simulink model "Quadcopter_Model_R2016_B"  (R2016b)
settings: Solver=VariableStepAuto  StartTime=0.0  StopTime=20  RelTol=1e-3
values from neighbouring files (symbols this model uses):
  g = 9.81    [modelParameters.m]
  If = 0.511    [modelParameters.m]
  Jreq = 4.2012e-05    [modelParameters.m]
  Jxx = 0.0218    [modelParameters.m]
  Jyy = 0.0277    [modelParameters.m]
  Jzz = 0.0332    [modelParameters.m]
  Kd = 1.8087e-07    [modelParameters.m]
  Kq = 96.3422    [modelParameters.m]
  Kt = 8.1558*10^-6    (= 8.1558e-06)    [modelParameters.m]
  Kv = 96.3422    [modelParameters.m]
  m = 1.19    [modelParameters.m]
  Pmax = 0.80    (= 0.8)    [modelParameters.m]
  Pmin = 0.40    (= 0.4)    [modelParameters.m]
  rhx = 0.016    [modelParameters.m]
  rhy = 0.016    [modelParameters.m]
  rhz = 0.003    [modelParameters.m]
  Rm = 0.2308    [modelParameters.m]
  Vb = 11.1    [modelParameters.m]
libraries: vrlib x2, simulink x2

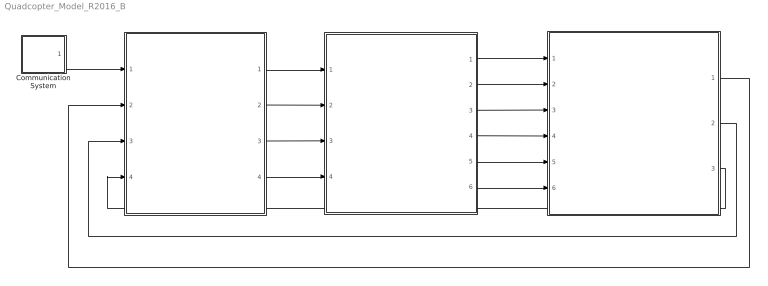
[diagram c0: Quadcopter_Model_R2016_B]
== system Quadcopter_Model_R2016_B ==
  " " : Subsystem
  "        " : Subsystem
  " " : Subsystem
  Communication System : Subsystem
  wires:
  " "/1(Rotor 0 Duty Cycle) -> " "/1(Rotor 0 Duty Cycle)
  "        "/2(euler_rates) -> " "/3(euler_rates)
  "        "/1(euler_angles_filtered) -> " "/2(euler_angles_filtered)
  Communication System/1(setpoints) -> " "/1(setpoints)
  " "/2(Rotor 1 Duty Cycle) -> " "/2(Rotor 1 Duty Cycle)
  " "/3(Rotor 2 Duty Cycle) -> " "/3(Rotor 2 Duty Cycle)
  " "/4(Rotor 3 Duty Cycle) -> " "/4(Rotor 3 Duty Cycle)
  " "/1(B_omega) -> "        "/1(B_Omega)
  " "/2(euler_angles) -> "        "/2(euler_angles)
  " "/3(B_vo) -> "        "/3(B_vo)
  " "/4(E_ro) -> "        "/4(E_ro)
  " "/5(B_vo_dot) -> "        "/5(B_vo_dot)
  " "/6(B_g) -> "        "/6(B_g)
  "        "/3(current_position) -> " "/4(current_position)

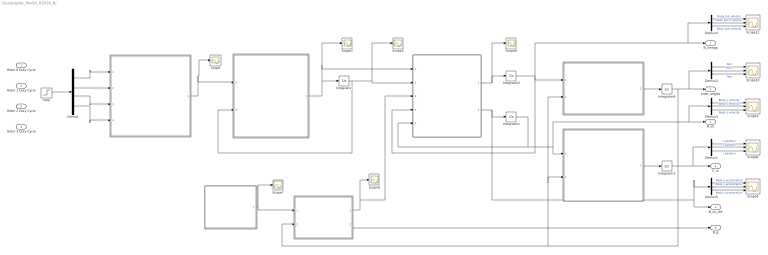
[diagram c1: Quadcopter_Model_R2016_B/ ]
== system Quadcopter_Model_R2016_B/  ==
  Rotor 0 Duty Cycle : Inport
  Rotor 1 Duty Cycle : Inport  Port=2
  Rotor 2 Duty Cycle : Inport  Port=3
  Rotor 3 Duty Cycle : Inport  Port=4
  " " : MATLAB Function  TreatAsAtomicUnit=on
  " " : MATLAB Function  TreatAsAtomicUnit=on
  " " : MATLAB Function  TreatAsAtomicUnit=on
  " " : MATLAB Function  TreatAsAtomicUnit=on
  " " : MATLAB Function  TreatAsAtomicUnit=on
  " " : MATLAB Function  TreatAsAtomicUnit=on
  " " : MATLAB Function  TreatAsAtomicUnit=on
  Demux : Demux
  Demux{1..5} (5 alike) : Demux  Outputs=3
  Integrator{,1..3} (4 alike) : Integrator
  Integrator4 : Integrator  ContinuousStateAttributes=['phi' 'theta' 'psi']
  Scope{,1..2,7..9} (6 alike) : Scope
  Scope{3..4,6,10..11} (5 alike) : Scope  NumInputPorts=3
  Step : Step  Before=68.25*ones(4,1)  After=[ 68.25; 69.25; 69.25; 68.25 ]  SampleTime=0
  B_omega : Outport
  euler_angles : Outport  Port=2
  B_vo : Outport  Port=3
  E_ro : Outport  Port=4
  B_vo_dot : Outport  Port=5
  B_g : Outport  Port=6
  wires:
  " "/1(Vb_eff) -> Scope/1, " "/1(Vb_eff)
  " "/1(angular_acceleration) -> Integrator/1, Scope1/1, " "/1(angular_acceleration)
  Integrator/1 -> Scope2/1, " "/2(angular_velocity), " "/2(angular_velocity)
  " "/1(B_omega_dot) -> Scope9/1, Integrator2/1
  " "/2(B_vo_dot) -> Demux5/1, B_vo_dot/1, Integrator1/1
  Integrator2/1 -> B_omega/1, Demux4/1, " "/4(B_omega), " "/1(B_omega)
  " "/1(euler_rates) -> Integrator4/1
  " "/1(E_Fg) -> Scope7/1, " "/1(E_Fg)
  " "/1(E_ro) -> Integrator3/1
  Integrator3/1 -> Demux1/1, E_ro/1
  " "/1(B_Fg) -> Scope8/1, " "/3(B_Fg)
  " "/2(B_g) -> B_g/1
  Demux/1 -> " "/1(rotor_0_duty_cycle)
  Demux/2 -> " "/2(rotor_1_duty_cycle)
  Demux/3 -> " "/3(rotor_2_duty_cycle)
  Demux/4 -> " "/4(rotor_3_duty_cycle)
  Step/1 -> Demux/1
  Demux1/2 -> Scope6/2  "y position"
  Demux1/1 -> Scope6/1  "x position"
  Demux1/3 -> Scope6/3  "z position"
  Integrator4/1 -> Demux2/1, euler_angles/1, " "/2(euler_angles), " "/2(euler_angles), " "/2(euler_angles)
  Demux2/2 -> Scope10/2  "Pitch"
  Demux2/1 -> Scope10/1  "Roll"
  Demux2/3 -> Scope10/3  "Yaw"
  Demux4/2 -> Scope11/2  "Body pitch velocity"
  Demux4/1 -> Scope11/1  "Body roll velocity"
  Demux4/3 -> Scope11/3  "Body yaw velocity"
  Demux3/2 -> Scope3/2  "Body y velocity"
  Demux3/1 -> Scope3/1  "Body x velocity"
  Demux3/3 -> Scope3/3  "Body z velocity"
  Demux5/2 -> Scope4/2  "Body y acceleration"
  Demux5/1 -> Scope4/1  "Body x acceleration"
  Demux5/3 -> Scope4/3  "Body z acceleration"
  Integrator1/1 -> " "/5(B_vo), " "/1(B_vo), Demux3/1, B_vo/1

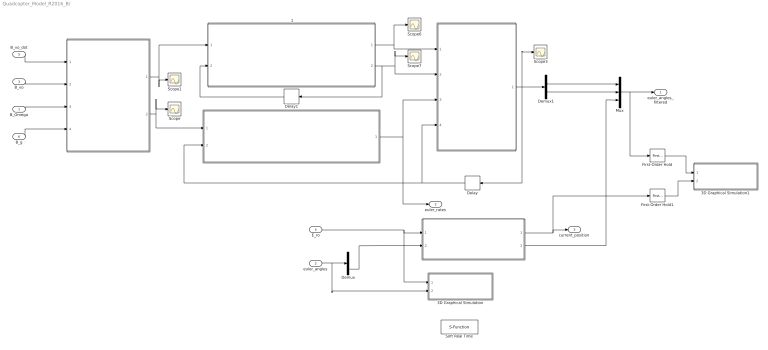
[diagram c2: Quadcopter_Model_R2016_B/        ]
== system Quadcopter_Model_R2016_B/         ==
  B_Omega : Inport
  euler_angles : Inport  Port=2
  B_vo : Inport  Port=3
  E_ro : Inport  Port=4
  B_vo_dot : Inport  Port=5
  B_g : Inport  Port=6
  " " : MATLAB Function  TreatAsAtomicUnit=on
  " " : Subsystem
  " " : MATLAB Function  TreatAsAtomicUnit=on
  " 1" : MATLAB Function  TreatAsAtomicUnit=on
  " " : Subsystem
  3D Graphical Simulation : Subsystem  Commented=on
  3D Graphical Simulation1 : Subsystem
  Delay : Delay  DelayLength=1  InitialCondition=0
  Delay1 : Delay  DelayLength=1  InitialCondition=0
  Demux : Demux  Outputs=3
  Demux1 : Demux  Outputs=2
  First-Order Hold : simulink/Discrete/First-Order Hold  DisableCoverage=on  Ts=6.1e-3
  First-Order Hold1 : simulink/Discrete/First-Order Hold  DisableCoverage=on  Ts=6.1e-3
  Mux : Mux  Inputs=3
  Scope{,1,3,6..7} (5 alike) : Scope
  Soft Real Time : S-Function  Commented=on  FunctionName=sfun_time  Parameters=x  SFunctionDeploymentMode=off  EnableBusSupport=off
  euler_angles_filtered : Outport
  euler_rates : Outport  Port=2
  current_position : Outport  Port=3
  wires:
  " "/1(accelerometer) -> " 1"/1(accel_reading), Scope1/1
  " "/2(gyroscope) -> Scope/1, " "/1(gyro_reading)
  B_vo_dot/1 -> " "/1(B_vo_dot)
  B_vo/1 -> " "/2(B_vo)
  B_Omega/1 -> " "/3(B_Omega)
  B_g/1 -> " "/4(B_g)
  " 1"/2(accel_roll) -> Delay1/1, " "/2(accel_roll), Scope7/1
  " 1"/1(accel_pitch) -> " "/1(accel_pitch), Scope6/1
  " "/1(euler_rates_IMU) -> euler_rates/1, " "/3(euler_angles_gyro)
  Delay/1 -> " "/4(prev_euler_angles_IMU), " "/2(euler_angles_IMU)
  Delay1/1 -> " 1"/2(accel_roll_prev)
  euler_angles/1 -> 3D Graphical Simulation/2(Euler Angles), Demux/1
  " "/1(euler_angles_IMU) -> Demux1/1, Delay/1, Scope3/1
  First-Order Hold/1 -> 3D Graphical Simulation1/1("Euler Angles ")
  E_ro/1 -> 3D Graphical Simulation/1(Displacement), " "/1(E_ro)
  Demux/3 -> " "/2(yaw)
  First-Order Hold1/1 -> 3D Graphical Simulation1/2(Displacement)
  Demux1/1 -> Mux/1
  Demux1/2 -> Mux/2
  " "/2(yaw_camera) -> Mux/3
  Mux/1 -> First-Order Hold/1, euler_angles_filtered/1
  " "/1(E_ro_camera) -> First-Order Hold1/1, current_position/1

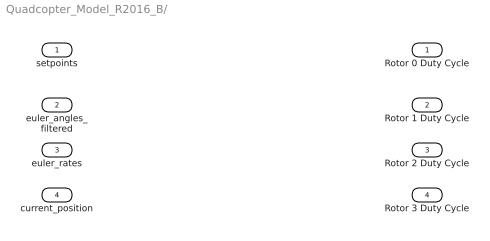
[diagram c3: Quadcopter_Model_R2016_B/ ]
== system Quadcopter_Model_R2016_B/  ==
  setpoints : Inport
  euler_angles_filtered : Inport  Port=2
  euler_rates : Inport  Port=3
  current_position : Inport  Port=4
  Rotor 0 Duty Cycle : Outport
  Rotor 1 Duty Cycle : Outport  Port=2
  Rotor 2 Duty Cycle : Outport  Port=3
  Rotor 3 Duty Cycle : Outport  Port=4

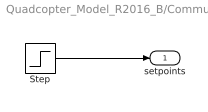
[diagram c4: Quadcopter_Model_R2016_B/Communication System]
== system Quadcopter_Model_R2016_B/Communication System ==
  Step : Step  Before=zeros(4,1)  After=[0; 0; 0; 0]  SampleTime=0
  setpoints : Outport
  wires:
  Step/1 -> setpoints/1

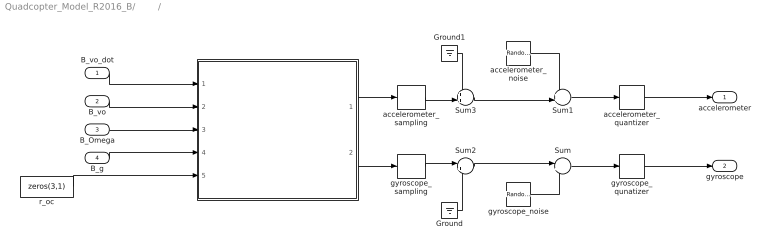
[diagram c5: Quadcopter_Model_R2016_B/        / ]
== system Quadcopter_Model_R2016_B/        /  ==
  B_vo_dot : Inport
  B_vo : Inport  Port=2
  B_Omega : Inport  Port=3
  B_g : Inport  Port=4
  " " : MATLAB Function  TreatAsAtomicUnit=on
  Ground : Ground
  Ground1 : Ground
  Sum : Sum  Inputs=|++
  Sum1 : Sum  Inputs=++|
  Sum2 : Sum  Inputs=|++
  Sum3 : Sum  Inputs=++|
  accelerometer_noise : RandomNumber  Mean=zeros(3,1)  Variance=[ 3e-7 ; 3.3e-7 ; 7.2e-7 ]  Seed=[0,1,2]  SampleTime=6.1e-3
  accelerometer_quantizer : Quantizer  QuantizationInterval=2.4400e-04
  accelerometer_sampling : ZeroOrderHold  SampleTime=6.1e-3
  gyroscope_noise : RandomNumber  Mean=zeros(3,1)  Variance=[ 2.2e-8 ; 1.1e-7 ; 2.4e-8 ]  Seed=[0,1,2]  SampleTime=6.1e-3
  gyroscope_qunatizer : Quantizer  QuantizationInterval=1.1e-3
  gyroscope_sampling : ZeroOrderHold  SampleTime=6.1e-3
  r_oc : Constant  Value=zeros(3,1)
  accelerometer : Outport
  gyroscope : Outport  Port=2
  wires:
  gyroscope_qunatizer/1 -> gyroscope/1
  accelerometer_quantizer/1 -> accelerometer/1
  accelerometer_noise/1 -> Sum1/1
  Sum/1 -> gyroscope_qunatizer/1
  Sum2/1 -> Sum/1
  Sum3/1 -> Sum1/2
  " "/2(gyroReading) -> gyroscope_sampling/1
  gyroscope_noise/1 -> Sum/2
  " "/1(accelReading) -> accelerometer_sampling/1
  Sum1/1 -> accelerometer_quantizer/1
  gyroscope_sampling/1 -> Sum2/1
  accelerometer_sampling/1 -> Sum3/2
  Ground/1 -> Sum2/2
  Ground1/1 -> Sum3/1
  B_vo_dot/1 -> " "/1(B_vo_dot)
  B_vo/1 -> " "/2(B_vo)
  B_Omega/1 -> " "/3(B_Omega)
  B_g/1 -> " "/4(B_g)
  r_oc/1 -> " "/5(r_oc)

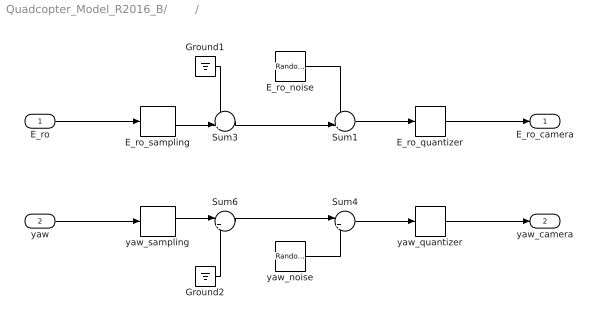
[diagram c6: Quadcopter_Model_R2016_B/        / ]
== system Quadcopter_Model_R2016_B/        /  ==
  E_ro : Inport
  yaw : Inport  Port=2
  E_ro_noise : RandomNumber  Mean=zeros(3,1)  Variance=[ 7.9664e-10 ; 1.1928e-10 ; 5.0636e-10 ]  Seed=[0,1,2]  SampleTime=6.1e-3
  E_ro_quantizer : Quantizer  QuantizationInterval=2.4400e-04
  E_ro_sampling : ZeroOrderHold  SampleTime=6.1e-3
  Ground1 : Ground
  Ground2 : Ground
  Sum1 : Sum  Inputs=++|
  Sum3 : Sum  Inputs=++|
  Sum4 : Sum  Inputs=|++
  Sum6 : Sum  Inputs=|++
  yaw_noise : RandomNumber  Variance=1.0783e-9  SampleTime=6.1e-3
  yaw_quantizer : Quantizer  QuantizationInterval=1.1e-3
  yaw_sampling : ZeroOrderHold  SampleTime=6.1e-3
  E_ro_camera : Outport
  yaw_camera : Outport  Port=2
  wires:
  E_ro_quantizer/1 -> E_ro_camera/1
  E_ro_noise/1 -> Sum1/1
  Sum3/1 -> Sum1/2
  Sum1/1 -> E_ro_quantizer/1
  E_ro_sampling/1 -> Sum3/2
  Ground1/1 -> Sum3/1
  yaw_quantizer/1 -> yaw_camera/1
  Sum4/1 -> yaw_quantizer/1
  Sum6/1 -> Sum4/1
  yaw_noise/1 -> Sum4/2
  yaw_sampling/1 -> Sum6/1
  Ground2/1 -> Sum6/2
  yaw/1 -> yaw_sampling/1
  E_ro/1 -> E_ro_sampling/1

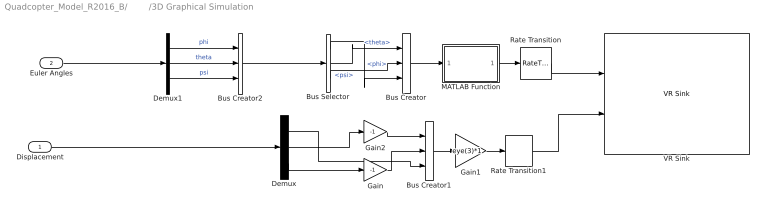
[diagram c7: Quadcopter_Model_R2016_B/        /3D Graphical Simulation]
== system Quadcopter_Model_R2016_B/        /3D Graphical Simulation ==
  Displacement : Inport
  Euler Angles : Inport  Port=2
  Bus Creator : BusCreator  Inputs=3
  Bus Creator1 : BusCreator  Inputs=3
  Bus Creator2 : BusCreator  Inputs=3
  Bus Selector : BusSelector  OutputSignals=phi,theta,psi
  Demux : Demux  Outputs=3
  Demux1 : Demux  Outputs=3
  Gain : Gain  Gain=-1
  Gain1 : Gain  Gain=eye(3)*1  Multiplication=Matrix(K*u)
  Gain2 : Gain  Gain=-1
  MATLAB Function : MATLAB Function  TreatAsAtomicUnit=on
  Rate Transition : RateTransition  OutPortSampleTime=0.06
  Rate Transition1 : RateTransition  OutPortSampleTime=0.06
  VR Sink : vrlib/VR Sink  InstantiateOnLoad=on  SampleTime=-1  ViewEnable=on  RemoteChange=off  RemoteView=off  FieldsWritten=Helicopter.rotation.4.1.1.double#Helicopter.translation.3.1.1.double  WorldFileName=quadrotor_world_ucart.wrl  AutoView=on  VideoDimensions=[]  AllowVariableSize=off
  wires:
  Displacement/1 -> Demux/1
  Bus Creator2/1 -> Bus Selector/1
  Demux/1 -> Bus Creator1/3
  Gain/1 -> Bus Creator1/2
  Gain2/1 -> Bus Creator1/1
  Rate Transition1/1 -> VR Sink/2
  Rate Transition/1 -> VR Sink/1
  Demux/3 -> Gain/1
  Demux/2 -> Gain2/1
  Bus Creator1/1 -> Gain1/1
  Bus Selector/1 -> Bus Creator/3  "<phi>"
  Bus Selector/3 -> Bus Creator/2  "<psi>"
  Bus Selector/2 -> Bus Creator/1  "<theta>"
  Gain1/1 -> Rate Transition1/1
  Demux1/3 -> Bus Creator2/3  "psi"
  Demux1/2 -> Bus Creator2/2  "theta"
  Demux1/1 -> Bus Creator2/1  "phi"
  Euler Angles/1 -> Demux1/1
  Bus Creator/1 -> MATLAB Function/1(u)
  MATLAB Function/1(y) -> Rate Transition/1

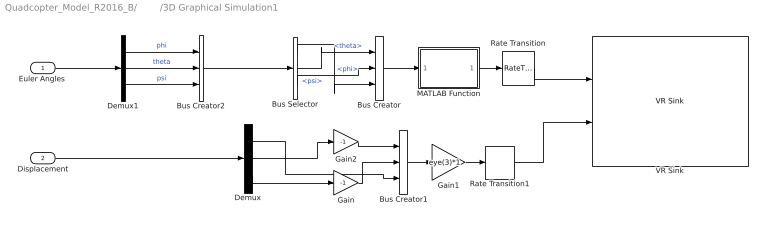
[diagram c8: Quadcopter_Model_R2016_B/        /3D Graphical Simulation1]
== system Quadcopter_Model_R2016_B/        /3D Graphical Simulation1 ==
  "Euler Angles " : Inport
  Displacement : Inport  Port=2
  Bus Creator : BusCreator  Inputs=3
  Bus Creator1 : BusCreator  Inputs=3
  Bus Creator2 : BusCreator  Inputs=3
  Bus Selector : BusSelector  OutputSignals=phi,theta,psi
  Demux : Demux  Outputs=3
  Demux1 : Demux  Outputs=3
  Gain : Gain  Gain=-1
  Gain1 : Gain  Gain=eye(3)*1  Multiplication=Matrix(K*u)
  Gain2 : Gain  Gain=-1
  MATLAB Function : MATLAB Function  TreatAsAtomicUnit=on
  Rate Transition : RateTransition  OutPortSampleTime=0.06
  Rate Transition1 : RateTransition  OutPortSampleTime=0.06
  VR Sink : vrlib/VR Sink  InstantiateOnLoad=on  SampleTime=-1  ViewEnable=on  RemoteChange=off  RemoteView=off  FieldsWritten=Helicopter.rotation.4.1.1.double#Helicopter.translation.3.1.1.double  WorldFileName=quadrotor_world_ucart.wrl  AutoView=on  VideoDimensions=[]  AllowVariableSize=off
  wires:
  Bus Creator2/1 -> Bus Selector/1
  Demux/1 -> Bus Creator1/3
  Gain/1 -> Bus Creator1/2
  Gain2/1 -> Bus Creator1/1
  Rate Transition1/1 -> VR Sink/2
  Rate Transition/1 -> VR Sink/1
  Demux/3 -> Gain/1
  Demux/2 -> Gain2/1
  Bus Creator1/1 -> Gain1/1
  Bus Selector/1 -> Bus Creator/3  "<phi>"
  Bus Selector/3 -> Bus Creator/2  "<psi>"
  Bus Selector/2 -> Bus Creator/1  "<theta>"
  Gain1/1 -> Rate Transition1/1
  Demux1/3 -> Bus Creator2/3  "psi"
  Demux1/2 -> Bus Creator2/2  "theta"
  Demux1/1 -> Bus Creator2/1  "phi"
  Bus Creator/1 -> MATLAB Function/1(u)
  MATLAB Function/1(y) -> Rate Transition/1
  Displacement/1 -> Demux/1
  "Euler Angles "/1 -> Demux1/1

== matlab function Quadcopter_Model_R2016_B/





/



 ==
function E_Fg = gravity(  m, g)

E_Fg = [0; 0; m*g];

== matlab function Quadcopter_Model_R2016_B/





/






 ==
function E_ro  = linear_body_earth_conversion(B_vo, euler_angles)

euler_rates = zeros(3,1);
E_ro = zeros(3,1);

phi = euler_angles(1);
theta = euler_angles(2);
psi = euler_angles(3);

Leb = [cos(theta)*cos(psi), sin(phi)*sin(theta)*cos(psi)-cos(phi)*sin(psi), cos(phi)*sin(theta)*cos(psi)+sin(phi)*sin(psi); ...
       cos(theta)*sin(psi), sin(phi)*sin(theta)*sin(psi)+cos(phi)*cos(psi), cos(phi)*sin(theta)*sin(psi)-sin(phi)*cos(psi); ...
           -sin(theta)    ,                sin(phi)*cos(theta)            ,                 cos(phi)*cos(theta)           ];

E_ro = Leb * B_vo;

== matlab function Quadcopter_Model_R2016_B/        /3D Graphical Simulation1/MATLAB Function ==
function y = eigenaxis_ucart(u)


if abs(u(1))< 0.0001
    u(1) = 0.0001;
end

if abs(u(2))< 0.0001
    u(2) = 0.0001;
end

if abs(u(3))< 0.0001
    u(3) = 0.0001;
end

u = [ -u(1); -u(2); u(3) ];% [Pitch, Yaw, Roll] 

C11 = cos(u(2))*cos(u(3));
C12 = cos(u(2))*sin(u(3));
C13 = -sin(u(2));
C21 = sin(u(1))*sin(u(2))*cos(u(3))-cos(u(1))*sin(u(3));
C22 = sin(u(1))*sin(u(2))*sin(u(3))+cos(u(1))*cos(u(3));
C23 = sin(u(1))*cos(u(2));
C31 = cos(u(1))*sin(u(2))*cos(u(3))+sin(u(1))*sin(u(3));
C32 = cos(u(1))*sin(u(2))*sin(u(3))-sin(u(1))*cos(u(3));
C33 = cos(u(1))*cos(u(2));
    
theta = acos(0.5*(C11+C22+C33-1));

e = [C23-C32; C31-C13; C12-C21]/(2*sin(theta));
    
y = [e; theta];

== matlab function Quadcopter_Model_R2016_B/





/

 ==
function Vb_eff   = ESC(rotor_0_duty_cycle, rotor_1_duty_cycle, rotor_2_duty_cycle, rotor_3_duty_cycle, Pmin, Pmax, Vb)

% Define u_Pi for each of the rotors
u_P0 = (rotor_0_duty_cycle/100 - Pmin) / (Pmax - Pmin);
u_P1 = (rotor_1_duty_cycle/100 - Pmin) / (Pmax - Pmin);
u_P2 = (rotor_2_duty_cycle/100 - Pmin) / (Pmax - Pmin);
u_P3 = (rotor_3_duty_cycle/100 - Pmin) / (Pmax - Pmin);

% Determine the effective battery voltage from each ESC
Vb_eff_0 = u_P0 * Vb;
Vb_eff_1 = u_P1 * Vb;
Vb_eff_2 = u_P2 * Vb;
Vb_eff_3 = u_P3 * Vb;

Vb_eff = [Vb_eff_0, Vb_eff_1, Vb_eff_2, Vb_eff_3];

== matlab function Quadcopter_Model_R2016_B/





/
 ==
function angular_acceleration  = motor(Vb_eff, angular_velocity, Rm, Kv, Kq, Kd, If, Jreq)

% Define each motors effective battery voltage
Vb_eff_0 = Vb_eff(1);
Vb_eff_1 = Vb_eff(2);
Vb_eff_2 = Vb_eff(3);
Vb_eff_3 = Vb_eff(4);

% Determine the angular velocity of each rotor from feedback
w_0 = angular_velocity(1);
w_1 = angular_velocity(2);
w_2 = angular_velocity(3);
w_3 = angular_velocity(4);

% Determine angular acceleration of each rotor
w_0_dot = 1/(Jreq*Rm*Kq) * Vb_eff_0 - 1/(Jreq*Rm*Kq*Kv) * w_0 - 1/(Jreq*Kq)*If - (Kd/Jreq) * w_0^2;
w_1_dot = 1/(Jreq*Rm*Kq) * Vb_eff_1 - 1/(Jreq*Rm*Kq*Kv) * w_1 - 1/(Jreq*Kq)*If - (Kd/Jreq) * w_1^2;
w_2_dot = 1/(Jreq*Rm*Kq) * Vb_eff_2 - 1/(Jreq*Rm*Kq*Kv) * w_2 - 1/(Jreq*Kq)*If - (Kd/Jreq) * w_2^2;
w_3_dot = 1/(Jreq*Rm*Kq) * Vb_eff_3 - 1/(Jreq*Rm*Kq*Kv) * w_3 - 1/(Jreq*Kq)*If - (Kd/Jreq) * w_3^2;

angular_acceleration = [w_0_dot, w_1_dot, w_2_dot, w_3_dot];

== matlab function Quadcopter_Model_R2016_B/





/







 ==
function [B_omega_dot, B_vo_dot]= rotor(angular_acceleration, angular_velocity, B_Fg, B_omega, B_vo, m, Kt, Kd, rhx, rhy, rhz, Jreq, Jxx, Jyy, Jzz)

B_vo_dot = zeros(3,1);
B_omega_dot = zeros(3,1);

% Create J vector
J = [Jxx,  0 ,  0 ; ...
      0 , Jyy,  0 ; ...
      0 ,  0 , Jzz;];

% Create r_hi vector
rh_0 = [-rhx; rhy; rhz];
rh_1 = [rhx; rhy; rhz];
rh_2 = [-rhx; -rhy; rhz];
rh_3 = [rhx; -rhy; rhz];

% Define vector from body frame origin to center of mass
br_oc = [0; 0; 0];

% Define 3x3 Identity Matrix
I = eye(3);

% Create gamma vectors
gamma_Ti = [0; 0; -1];
gamma_omega_03 = [0; 0; -1];  %Rotors 0 and 3 use this gamma_omega vector
gamma_omega_12 = [0; 0; 1]; %Rotors 1 and 2 use this gamma_omega vector

% Define angular velocities for each rotor
w_0 = angular_velocity(1);
w_1 = angular_velocity(2);
w_2 = angular_velocity(3);
w_3 = angular_velocity(4);

% Define angular acceleration for each rotor
w_0_dot = angular_acceleration(1);
w_1_dot = angular_acceleration(2);
w_2_dot = angular_acceleration(3);
w_3_dot = angular_acceleration(4);

% Define the rotor force in the z-direction from each rotor
B_Fr_0 = Kt * w_0 * w_0 * gamma_Ti;
B_Fr_1 = Kt * w_1 * w_1 * gamma_Ti;
B_Fr_2 = Kt * w_2 * w_2 * gamma_Ti;
B_Fr_3 = Kt * w_3 * w_3 * gamma_Ti;

% Sum up the rotor forces in the z-direction from each vector to get the
% total body force in the z-direction
B_Fr = B_Fr_0 + B_Fr_1 + B_Fr_2 + B_Fr_3;

% Define the in-plane drag and induced torque produced by each rotor
 B_Q_d0 = -1 * Kd * w_0 * w_0 * gamma_omega_03;
 B_Q_d1 = -1 * Kd * w_1 * w_1 * gamma_omega_12;
 B_Q_d2 = -1 * Kd * w_2 * w_2 * gamma_omega_12;
 B_Q_d3 = -1 * Kd * w_3 * w_3 * gamma_omega_03;

% Sum up the total in-plane drag and induced torque to get the total
% in-plane drag and induced torque on the body
B_Q_d = B_Q_d0 + B_Q_d1 + B_Q_d2 + B_Q_d3;

% Define the force lever arm torque created from the force produced by each
% rotor in the z-direction
B_Q_F0 = cross( rh_0, B_Fr_0 );
B_Q_F1 = cross( rh_1, B_Fr_1 );
B_Q_F2 = cross( rh_2, B_Fr_2 );
B_Q_F3 = cross( rh_3, B_Fr_3 );

B_Q_F = B_Q_F0 + B_Q_F1 + B_Q_F2 + B_Q_F3;

%Define the change in angular momentum torque produced by each rotor 
B_Q_L0 = -1 * Jreq * ( cross(B_omega, w_0 * gamma_omega_03) + w_0_dot * gamma_omega_03 );
B_Q_L1 = -1 * Jreq * ( cross(B_omega, w_1 * gamma_omega_12) + w_1_dot * gamma_omega_12 ); 
B_Q_L2 = -1 * Jreq * ( cross(B_omega, w_2 * gamma_omega_12) + w_2_dot * gamma_omega_12 ); 
B_Q_L3 = -1 * Jreq * ( cross(B_omega, w_3 * gamma_omega_03) + w_3_dot * gamma_omega_03 );

% Sum up the total change in angular momentum torque produced by each rotor
B_Q_L = B_Q_L0 + B_Q_L1 + B_Q_L2 + B_Q_L3;

% Define the total rotor system torque as the sum of the in-plane drag and
% induced torque, force lever arm torque, and change in angular momentum
% torques
B_Q = B_Q_d + B_Q_F + B_Q_L;

% Define the body forces in the z-direction from each vector to get the
% total body force in the z-direction
B_F = B_Fr + B_Fg; 

% Define the body frame linear velocities
B_vo_dot = (m*I)^(-1) * ( B_F - cross( B_omega, m*(B_vo + cross(B_omega, br_oc)) ) );

% Define the body frame angular velocities
B_omega_dot = J ^(-1) * ( B_Q - cross(B_omega, J * B_omega) - cross(br_oc, B_F) );

== matlab function Quadcopter_Model_R2016_B/





/














 ==
function euler_rates = angular_body_earth_conversion(B_omega, euler_angles)

euler_rates = zeros(3,1);

phi = euler_angles(1);
theta = euler_angles(2);

Aeb = [1, sin(phi)*tan(theta), cos(phi)*tan(theta); ...
       0,     cos(phi)       ,        -sin(phi)   ; ...
       0,  sin(phi)/cos(theta), cos(phi)/cos(theta)];

   
euler_rates = Aeb * B_omega;

== matlab function Quadcopter_Model_R2016_B/





/






















 ==
function [B_Fg, B_g]  = linear_earth_body_conversion(E_Fg, euler_angles, m)

phi = euler_angles(1);
theta = euler_angles(2);
psi = euler_angles(3);

Lbe = [             cos(theta)*cos(psi)              ,          cos(theta)*sin(psi)                  ,     -sin(theta)    ; ...
       sin(phi)*sin(theta)*cos(psi)-cos(phi)*sin(psi), sin(phi)*sin(theta)*sin(psi)+cos(phi)*cos(psi), sin(phi)*cos(theta); ...
       cos(phi)*sin(theta)*cos(psi)+sin(phi)*sin(psi), cos(phi)*sin(theta)*sin(psi)-sin(phi)*cos(psi), cos(phi)*cos(theta)];

B_Fg = Lbe * E_Fg;

B_g = B_Fg/m;

== matlab function Quadcopter_Model_R2016_B/        /







 ==
function euler_angles_IMU  = complimentaryFilter(accel_pitch, accel_roll, euler_angles_gyro, prev_euler_angles_IMU)

LOOP_TIME = 6.1*10^-3;

prev_phi = prev_euler_angles_IMU(1);
prev_theta = prev_euler_angles_IMU(2);

phi_dot_gyro = euler_angles_gyro(1);
theta_dot_gyro = euler_angles_gyro(2);

phi = 0.98 * (prev_phi + phi_dot_gyro * LOOP_TIME ) + 0.02 * accel_roll;
theta = 0.98 * (prev_theta + theta_dot_gyro * LOOP_TIME) + 0.02 * accel_pitch;

euler_angles_IMU = [phi; theta];

== matlab function Quadcopter_Model_R2016_B/        /









/






 ==
function [accelReading,gyroReading] = idealIMU(B_vo_dot, B_vo, B_Omega, B_g, r_oc, g)
%#codegen

a = B_vo_dot + cross(B_Omega,B_vo) ; % body frame acceleration 

accelReading = (a - B_g)/g ; % accelerometer reading (ideal)

gyroReading = B_Omega ; % gyroscope reading (ideal) 

end

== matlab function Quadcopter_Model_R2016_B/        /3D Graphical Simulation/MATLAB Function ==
function y = eigenaxis_ucart(u)


if abs(u(1))< 0.0001
    u(1) = 0.0001;
end

if abs(u(2))< 0.0001
    u(2) = 0.0001;
end

if abs(u(3))< 0.0001
    u(3) = 0.0001;
end

u = [ -u(1); -u(2); u(3) ];% [Pitch, Yaw, Roll] 

C11 = cos(u(2))*cos(u(3));
C12 = cos(u(2))*sin(u(3));
C13 = -sin(u(2));
C21 = sin(u(1))*sin(u(2))*cos(u(3))-cos(u(1))*sin(u(3));
C22 = sin(u(1))*sin(u(2))*sin(u(3))+cos(u(1))*cos(u(3));
C23 = sin(u(1))*cos(u(2));
C31 = cos(u(1))*sin(u(2))*cos(u(3))+sin(u(1))*sin(u(3));
C32 = cos(u(1))*sin(u(2))*sin(u(3))-sin(u(1))*cos(u(3));
C33 = cos(u(1))*cos(u(2));
    
theta = acos(0.5*(C11+C22+C33-1));

e = [C23-C32; C31-C13; C12-C21]/(2*sin(theta));
    
y = [e; theta];

== matlab function Quadcopter_Model_R2016_B/        /














 ==
function euler_rates_IMU = angular_body_earth_conversion(gyro_reading, euler_angles_IMU)

phi = euler_angles_IMU(1);
theta = euler_angles_IMU(2);

Aeb = [1, sin(phi)*tan(theta), cos(phi)*tan(theta); ...
       0,     cos(phi)       ,        -sin(phi)   ; ...
       0,  sin(phi)/cos(theta), cos(phi)/cos(theta)];

   
euler_rates_IMU = Aeb * gyro_reading;

== matlab function Quadcopter_Model_R2016_B/        /











1 ==
function [accel_pitch, accel_roll] = getPitchAndRoll(accel_reading, accel_roll_prev)

mag = norm(accel_reading);

x_accel = accel_reading(1)/mag;
y_accel = accel_reading(2)/mag;
z_accel = accel_reading(3)/mag;

accel_pitch = atan(x_accel/sqrt(y_accel^2 + z_accel^2));
%unwrapped_pitch = unwrap([accel_pitch_prev accel_pitch]);
%accel_pitch = unwrapped_pitch(2);

accel_roll = atan2( -y_accel,(sign(-z_accel)*sqrt(z_accel^2 + (1/100)*x_accel^2)) );
unwrapped_roll = unwrap([accel_roll_prev accel_roll]);
accel_roll = unwrapped_roll(2);
